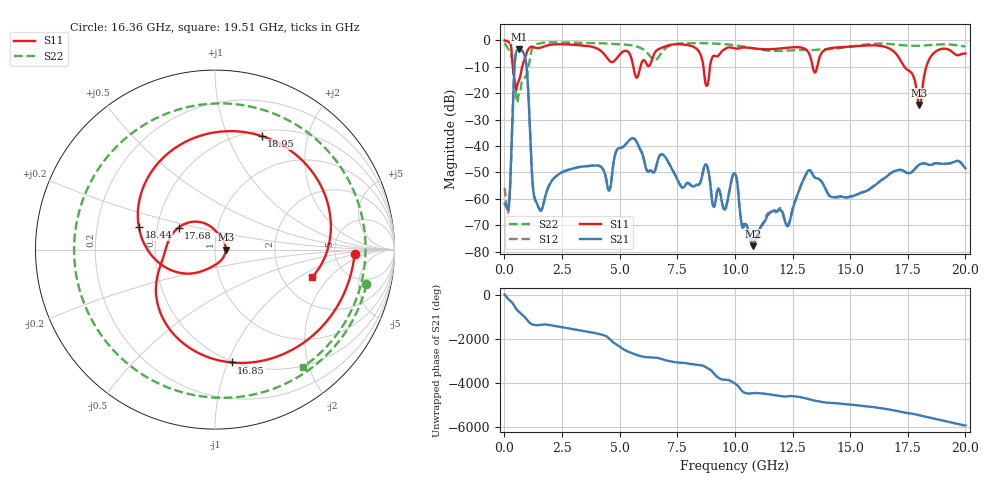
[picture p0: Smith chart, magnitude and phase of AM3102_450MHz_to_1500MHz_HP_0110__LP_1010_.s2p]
!Agilent Technologies,E8364B,MY43040894,A.07.50.67
!Agilent E8364B: A.07.50.67
!Date: Thursday, January 11, 2018 05:48:54
!Correction: S11(Full 2 Port(1,2))
!S21(Full 2 Port(1,2))
!S12(Full 2 Port(1,2))
!S22(Full 2 Port(1,2))
!S2P File: Measurements: S11, S21, S12, S22:
# Hz S  dB  R 50
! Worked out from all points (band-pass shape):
!   1601 points, 10 MHz to 20 GHz, reference 50 ohm
!   highest |S21| = -3.38 dB at 634.7 MHz (marker M1); lowest = -77.9 dB at 10.8 GHz (marker M2)
!   |S21| within 3 dB of the highest: 472.9 MHz to 892.8 MHz (419.9 MHz wide, 61.5 % of centre)
!   lowest |S11| = -24.5 dB at 18 GHz (marker M3), VSWR 1.13, Z = 56.4 + j0.00697 ohm
!   |S11| at or under -10 dB: 367.2 MHz to 773 MHz (405.8 MHz wide, 71.2 % of centre); 5.595 GHz to 5.901 GHz (305.4 MHz wide, 5.31 % of centre); 17.35 GHz to 18.31 GHz (951.5 MHz wide, 5.34 % of centre)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
!   |S22| runs from -23.6 to -0.8 dB; largest |S21 - S12| = 0.0022
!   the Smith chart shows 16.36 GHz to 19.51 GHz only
!   S11 on the Smith chart (normalised r, x): 16.36 GHz: 7.91, -0.92; 16.85 GHz: 0.49, -1.03; 17.68 GHz: 0.65, +0.17; 18.44 GHz: 0.39, +0.12; 18.95 GHz: 0.56, +1.33; 19.51 GHz: 2.90, -1.32
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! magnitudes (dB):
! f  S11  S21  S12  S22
! 10 MHz  -0.1  -61.8  -55.8  -1.1
! 197.4 MHz  -0.7  -62.3  -63.0  -3.6
! 447.3 MHz  -15.4  -8.9  -8.9  -16.1
! 634.7 MHz  -15.1  -3.4  -3.4  -20.3
! 934.5 MHz  -5.5  -8.1  -8.1  -13.5
! 1.247 GHz  -2.5  -56.2  -56.1  -2.5
! 1.484 GHz  -2.9  -63.2  -63.2  -1.3
! 3.346 GHz  -2.0  -47.8  -47.8  -1.0
! 6.682 GHz  -3.4  -44.7  -44.7  -6.4
! 9.543 GHz  -3.5  -64.0  -64.0  -1.5
! 10.01 GHz  -3.1  -50.5  -50.4  -1.9
! 10.8 GHz  -3.0  -77.9  -76.5  -3.0
! 13.34 GHz  -8.6  -50.2  -50.2  -3.7
! 16.36 GHz  -2.2  -52.8  -52.9  -1.3
! 16.68 GHz  -3.0  -50.8  -50.8  -1.4
! 16.85 GHz  -3.9  -49.8  -49.9  -1.5
! 17.68 GHz  -12.5  -49.8  -49.9  -2.1
! 18 GHz  -24.5  -47.0  -47.1  -2.1
! 18.44 GHz  -7.1  -47.1  -47.2  -1.8
! 18.95 GHz  -3.3  -46.7  -46.7  -1.5
! 19.51 GHz  -5.0  -46.0  -46.0  -1.8
! 20 GHz  -5.0  -48.4  -48.4  -2.3
